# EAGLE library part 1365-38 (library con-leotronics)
DUAL ROW STRAIGHT HEADER 1364 SERIES. 1.27mm x 1.27mm. Without Fixing Post. SMT Source: http://www.leotronics.co.uk/Conexcon/Data%20Sheets/sec.%20A/1364ing.pdf
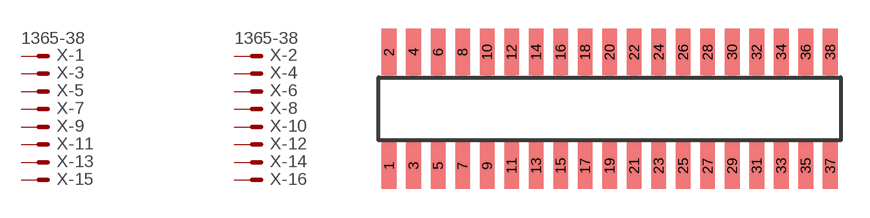
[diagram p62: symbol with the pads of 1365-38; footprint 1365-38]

Designator prefix X; gates -1=MVAL -2=MVAL -3=M -4=M -5=M -6=M -7=M -8=M -9=M -10=M -11=M -12=M -13=M -14=M -15=M -16=M -17=M -18=M -19=M -20=M -21=M -22=M -23=M -24=M -25=M -26=M -27=M -28=M -29=M -30=M -31=M -32=M -33=M -34=M -35=M -36=M -37=M -38=M

## 1365-38 (OC_FARNELL: unknown; OC_NEWARK: unknown)  [1365-38]
1  -1:S  pas
2  -2:S  pas
3  -3:S  pas
4  -4:S  pas
5  -5:S  pas
6  -6:S  pas
7  -7:S  pas
8  -8:S  pas
9  -9:S  pas
10  -10:S  pas
11  -11:S  pas
12  -12:S  pas
13  -13:S  pas
14  -14:S  pas
15  -15:S  pas
16  -16:S  pas
17  -17:S  pas
18  -18:S  pas
19  -19:S  pas
20  -20:S  pas
21  -21:S  pas
22  -22:S  pas
23  -23:S  pas
24  -24:S  pas
25  -25:S  pas
26  -26:S  pas
27  -27:S  pas
28  -28:S  pas
29  -29:S  pas
30  -30:S  pas
31  -31:S  pas
32  -32:S  pas
33  -33:S  pas
34  -34:S  pas
35  -35:S  pas
36  -36:S  pas
37  -37:S  pas
38  -38:S  pas

## Footprint 1365-38 (pad centres in mm)
DUAL ROW STRAIGHT HEADER 1364 SERIES. 1.27mm x 1.27mm. Without Fixing Post. SMT Source: http://www.leotronics.co.uk/Conexcon/Data%20Sheets/sec.%20A/1364ing.pdf
smd 0.76 x 2.4: 1 -11.43,-2.95; 2 -11.43,2.95; 3 -10.16,-2.95; 4 -10.16,2.95; 5 -8.89,-2.95; 6 -8.89,2.95; 7 -7.62,-2.95; 8 -7.62,2.95; 9 -6.35,-2.95; 10 -6.35,2.95; 11 -5.08,-2.95; 12 -5.08,2.95; 13 -3.81,-2.95; 14 -3.81,2.95; 15 -2.54,-2.95; 16 -2.54,2.95; 17 -1.27,-2.95; 18 -1.27,2.95; 19 0,-2.95; 20 0,2.95; 21 1.27,-2.95; 22 1.27,2.95; 23 2.54,-2.95; 24 2.54,2.95; 25 3.81,-2.95; 26 3.81,2.95; 27 5.08,-2.95; 28 5.08,2.95; 29 6.35,-2.95; 30 6.35,2.95; 31 7.62,-2.95; 32 7.62,2.95; 33 8.89,-2.95; 34 8.89,2.95; 35 10.16,-2.95; 36 10.16,2.95; 37 11.43,-2.95; 38 11.43,2.95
